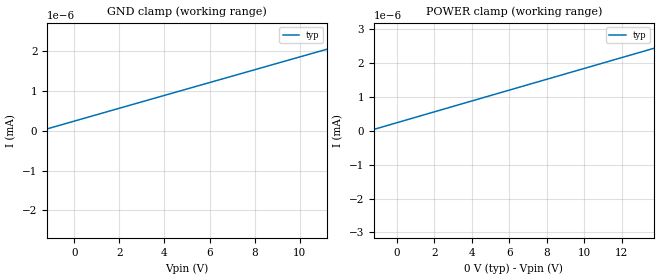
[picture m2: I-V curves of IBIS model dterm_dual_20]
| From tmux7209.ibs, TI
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| dterm_dual_20
[Model]   dterm_dual_20
Model_type   Terminator
|   typ   min   max
C_comp   4.014581e-11   NA   NA
[Voltage Range]   0   -20   20
[Temperature Range]   27   NA   NA
[Power Clamp Reference]   0   NA   NA
[GND Clamp Reference]   0   NA   NA
[GND Clamp]
|   Voltage   I(typ)   I(min)   I(max)
-25V      -4.62A     NA         NA
-17.27V   -2.585nA   NA         NA
-3.636V   -351.8pA   NA         NA
14.55V    2.57nA     NA         NA
20V       3.449nA    NA         NA
[POWER Clamp]
|   Voltage   I(typ)   I(min)   I(max)
-20V      -3.042nA   NA         NA
-5V       -572.8pA   NA         NA
17.27V    3.007nA    NA         NA
17.73V    3.08nA     NA         NA
25V       5.414A     NA         NA
